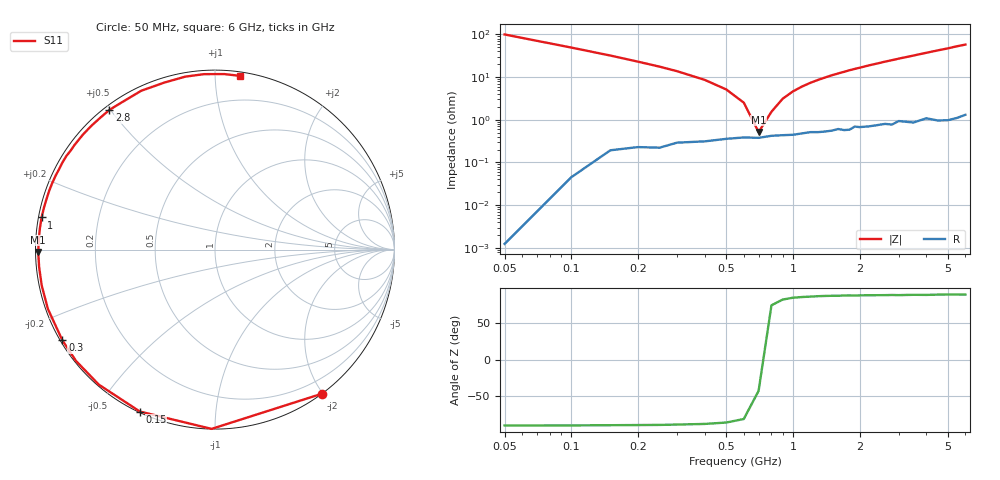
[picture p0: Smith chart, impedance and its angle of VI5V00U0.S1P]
! Infineon Technologies  Discrete & RF Semiconductors
! BB 804
! Si Tuning Diode in SOT23
! VR = 5 V
! S-Parameters:  July  1999
# GHz  S  MA  R  50
!  f  S11
! GHz  MAG  ANG
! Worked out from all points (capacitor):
!   34 points, 50 MHz to 6 GHz, reference 50 ohm
!   read as one part to ground: C = 31.8 pF near 50 MHz
!   lowest |Z| = 514 mohm at 700 MHz (marker M1)
!   series resonance near 719 MHz, so ESL is about 1.5 nH
!   S11 on the Smith chart (normalised r, x): 50 MHz: 0.00, -1.99; 150 MHz: 0.00, -0.64; 300 MHz: 0.01, -0.27; 1 GHz: 0.01, +0.09; 2.8 GHz: 0.02, +0.50; 6 GHz: 0.03, +1.15
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0.05  1 -53.4
0.1  0.9991 -91.1
0.15  0.9945 -114.9
0.2  0.9925 -130.7
0.25  0.9921 -141.3
0.3  0.9892 -149.3
0.4  0.9879 -160.5
0.5  0.9859 -168.3
0.6  0.9847 -174.3
0.7  0.985 -179.2
0.8  0.9833 176.6
1  0.9825 169.5
1.1  0.9813 166.3
1.3  0.9802 160.5
1.5  0.9789 155.1
1.6  0.9773 152.7
1.9  0.975 145.5
2.2  0.9757 138.9
2.4  0.9748 134.9
2.6  0.9739 130.7
2.8  0.9755 127.1
3  0.9715 123.3
3.5  0.9758 114.9
4  0.9724 106.9
4.5  0.9777 99.8
5  0.9795 93.6
5.5  0.9793 87.0
6  0.9778 81.9
